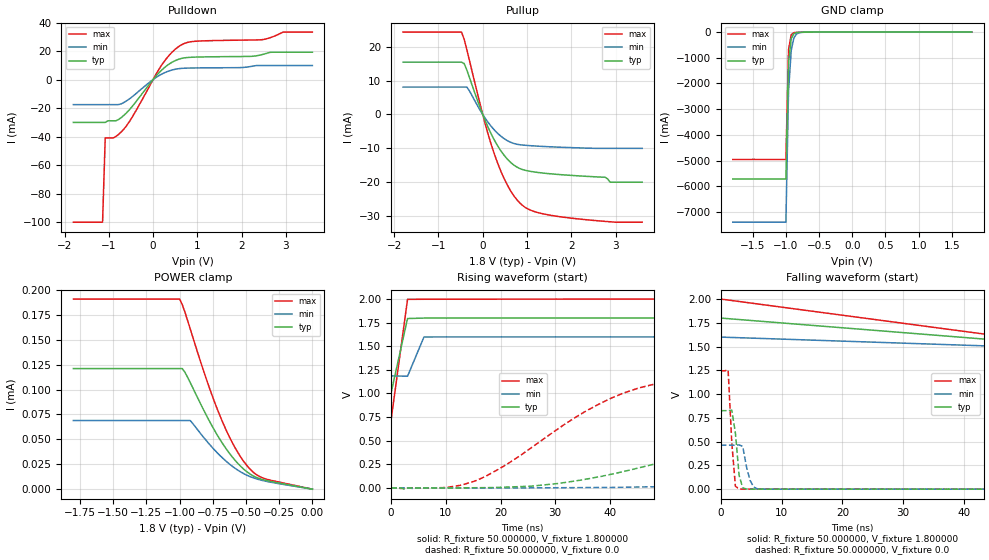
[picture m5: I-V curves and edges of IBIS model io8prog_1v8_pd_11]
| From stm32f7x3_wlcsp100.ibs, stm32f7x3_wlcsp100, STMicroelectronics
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|   Model io8prog_1v8_pd_11
[Model]  io8prog_1v8_pd_11
Model_type I/O
Polarity   Non-Inverting
Enable   Active-Low
Vinl =   0.540000V
Vinh =   1.260000V
Vmeas =  0.900000V
Cref =   100.000000nF
Rref =   1.000000k
Vref =   1.800000V
C_comp   2.595400pF   2.437600pF   2.808600pF
[Temperature Range]   25.000000   0.125000k   -40.000000
[Pullup Reference]   1.800000V   1.600000V   2.000000V
[Pulldown Reference]   0.0V   0.0V   0.0V
[POWER Clamp Reference]   1.800000V   1.600000V   2.000000V
[GND Clamp Reference]   0.0V   0.0V   0.0V
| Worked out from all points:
|   slope of the pulldown table from 0 to 0.27 V, typ, clamps not added: 31 ohm
|   slope of the pullup table from 0 to 0.27 V, typ, clamps not added: 34.9 ohm
|   GND clamp passes 1 mA (typ) near -0.57 V on its own axis
|   rising waveform, R_fixture 50.000000, V_fixture 1.800000: 20-80 % time 1.82ns typ, 1.79ns min, 1.81ns max; typ from 1.01 V to 1.8 V
|   rising waveform, R_fixture 50.000000, V_fixture 0.0: 20-80 % time 42.7ns typ, 82.4ns min, 21ns max; typ from 0 V to 0.826 V
|   falling waveform, R_fixture 50.000000, V_fixture 1.800000: 20-80 % time 93.2ns typ, 131ns min, 90.3ns max; typ from 1.8 V to 1.01 V
|   falling waveform, R_fixture 50.000000, V_fixture 0.0: 20-80 % time 755ps typ, 980ps min, 713ps max; typ from 0.826 V to 0 V
[Pulldown]
|Voltage   I(typ)   I(min)   I(max)
-1.8V     -30mA      -17.52mA   -100mA
-1.14V    -30mA      -17.52mA   -100mA
-1.08V    -30mA      -17.52mA   -40.9mA
-840mV    -28.88mA   -17.52mA   -39.94mA
-600mV    -23.35mA   -14.94mA   -32.45mA
180mV     6.236mA    3.598mA    9.492mA
540mV     13.85mA    7.499mA    22.29mA
720mV     15.32mA    8.029mA    25.55mA
900mV     15.74mA    8.167mA    26.76mA
2.46V     17.54mA    9.893mA    28.01mA
2.94V     19.23mA    9.893mA    33.35mA
3.6V      19.23mA    9.893mA    33.35mA
[Pullup]
|Voltage   I(typ)   I(min)   I(max)
-1.8V     15.46mA    8.1mA      24.33mA
-480mV    15.46mA    8.1mA      24.33mA
-360mV    13.15mA    8.1mA      19.18mA
60mV      -1.95mA    -1.198mA   -2.977mA
300mV     -8.441mA   -5.092mA   -13.07mA
600mV     -13.78mA   -8.025mA   -21.88mA
900mV     -16.27mA   -9.02mA    -26.86mA
1.2V      -17.03mA   -9.318mA   -28.8mA
1.74V     -17.74mA   -9.658mA   -30.18mA
2.76V     -18.5mA    -10mA      -31.55mA
2.88V     -20mA      -10mA      -31.68mA
3.6V      -20mA      -10mA      -31.8mA
[GND_clamp]
|Voltage   I(typ)   I(min)   I(max)
-1.8V     -5.722A    -7.401A    -4.956A
-1V       -5.722A    -7.401A    -4.956A
-960mV    -1.203A    -2.294A    -680.3mA
-920mV    -260.8mA   -717.4mA   -103.7mA
-880mV    -62.28mA   -228.9mA   -23.86mA
-840mV    -19.06mA   -76.33mA   -11.32mA
-760mV    -5.585mA   -11.67mA   -6.214mA
-640mV    -2.06mA    -2.422mA   -2.211mA
1.8V      44.31uA    33.68uA    51.4uA
[POWER_clamp]
|Voltage   I(typ)   I(min)   I(max)
-1.8V     121uA      68.85uA    190.7uA
-1V       121uA      68.85uA    190.7uA
-980mV    121uA      68.85uA    185.3uA
-960mV    117.4uA    68.85uA    177.7uA
-920mV    107uA      68.85uA    160.9uA
-800mV    74.53uA    48.91uA    111uA
-720mV    55.17uA    36.99uA    81.65uA
-620mV    35.16uA    24.73uA    51.11uA
-520mV    20.42uA    15.79uA    28.41uA
-440mV    12.93uA    11.16uA    16.44uA
-380mV    9.841uA    8.859uA    11.63uA
0V        0A         11.03nA    0A
[Ramp]
| variable   typ   min   max
dV/dt_r  0.49533/42.68723n   0.27782/83.69974n   0.74670/20.99069n
dV/dt_f  0.47520/41.75159n   0.24786/72.96807n   0.76679/23.30881n
R_load = 50.000000
[Rising Waveform]
R_fixture= 50.000000
V_fixture= 1.800000
V_fixture_min= 1.600000
V_fixture_max= 2.000000
|time   V(typ)   V(min)   V(max)
0s        1.007V     1.186V     721.4mV
3.003ns   1.793V     1.183V     1.996V
6.006ns   1.798V     1.598V     1.997V
297.3ns   1.799V     1.599V     1.999V
[Rising Waveform]
R_fixture= 50.000000
V_fixture= 0.0
V_fixture_min= 0.0
V_fixture_max= 0.0
|time   V(typ)   V(min)   V(max)
0s        195.6uV    220.2uV    196.3uV
15.02ns   1.982mV    442.3uV    67.53mV
30.03ns   43.95mV    2.116mV    606.9mV
40.24ns   145mV      5.355mV    951.1mV
49.25ns   268.7mV    13.57mV    1.115V
60.66ns   424.6mV    29.45mV    1.196V
86.49ns   673.8mV    107.9mV    1.238V
115.9ns   783mV      226.2mV    1.244V
192.2ns   823.2mV    414.1mV    1.245V
299.1ns   825.7mV    463.3mV    1.245V
[Falling Waveform]
R_fixture= 50.000000
V_fixture= 1.800000
V_fixture_min= 1.600000
V_fixture_max= 2.000000
|time   V(typ)   V(min)   V(max)
0s        1.799V     1.599V     1.999V
150.2ns   1.034V     1.281V     723.8mV
300.3ns   1.008V     1.193V     721.4mV
450.5ns   1.007V     1.187V     721.4mV
14.86us   1.007V     1.186V     721.4mV
[Falling Waveform]
R_fixture= 50.000000
V_fixture= 0.0
V_fixture_min= 0.0
V_fixture_max= 0.0
|time   V(typ)   V(min)   V(max)
0s        825.7mV    463.3mV    1.245V
1.201ns   825.4mV    463.3mV    1.254V
1.802ns   830.9mV    463.3mV    491.1mV
2.402ns   588.1mV    462.6mV    29.97mV
3.003ns   147.2mV    465.9mV    2.589mV
3.604ns   13.64mV    449.9mV    1.051mV
4.805ns   938.3uV    93.4mV     939.8uV
5.405ns   729.1uV    22.13mV    932.7uV
6.607ns   678uV      1.506mV    924.8uV
299.1ns   195.6uV    220.2uV    196.3uV
